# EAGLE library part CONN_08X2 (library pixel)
Multi connection point. Often used as Generic Header-pin footprint for 0.1 inch spaced/style header connections For AVR SPI programming port, see special device with nice symbol: "AVR_SPI_PROG_5x2.dev" You can populate with any combo of single row headers, but if you'd like an exact match, check these: 2x5 AVR ICSP Male Header (PRT-00778) 2x5 Pin Shrouded Header (PRT-08506) On any of the 0.1 inch spaced packages, you can populate with these: Break Away Headers - Straight (PRT-00116) Break Away Male Headers - Right Angle (PRT-00553) Female Headers (PRT-00115) Break Away Headers - Machine Pin (PRT-00117) Break Away Female Headers - Swiss Machine Pin (PRT-00743) Special note: the shrouded connector mates well with our 5x2 ribbon cables: 2x5 Pin IDC Ribbon Cable (PRT-08535)
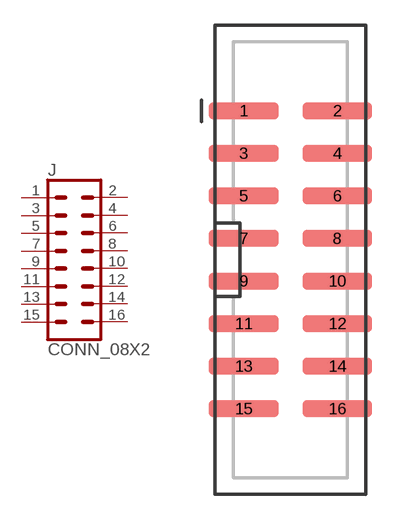
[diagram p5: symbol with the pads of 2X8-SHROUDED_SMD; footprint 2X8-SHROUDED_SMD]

Designator prefix J

## CONN_08X2SHD_SMD (PROD_ID: CONN-09508)  [2X8-SHROUDED_SMD]
1  1  pas
2  2  pas
3  3  pas
4  4  pas
5  5  pas
6  6  pas
7  7  pas
8  8  pas
9  9  pas
10  10  pas
11  11  pas
12  12  pas
13  13  pas
14  14  pas
15  15  pas
16  16  pas

## Footprint 2X8-SHROUDED_SMD (pad centres in mm)
Surface Mount - 2x5 Shrouded Header Specifications: Pin count:10 Pin pitch:0.1" Datasheet referenced for footprint Example device(s): CONN_05x2
smd 4.15 x 1: 1 -2.794,8.89; 2 2.794,8.89; 3 -2.794,6.35; 4 2.794,6.35; 5 -2.794,3.81; 6 2.794,3.81; 7 -2.794,1.27; 8 2.794,1.27; 9 -2.794,-1.27; 10 2.794,-1.27; 11 -2.794,-3.81; 12 2.794,-3.81; 13 -2.794,-6.35; 14 2.794,-6.35; 15 -2.794,-8.89; 16 2.794,-8.89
